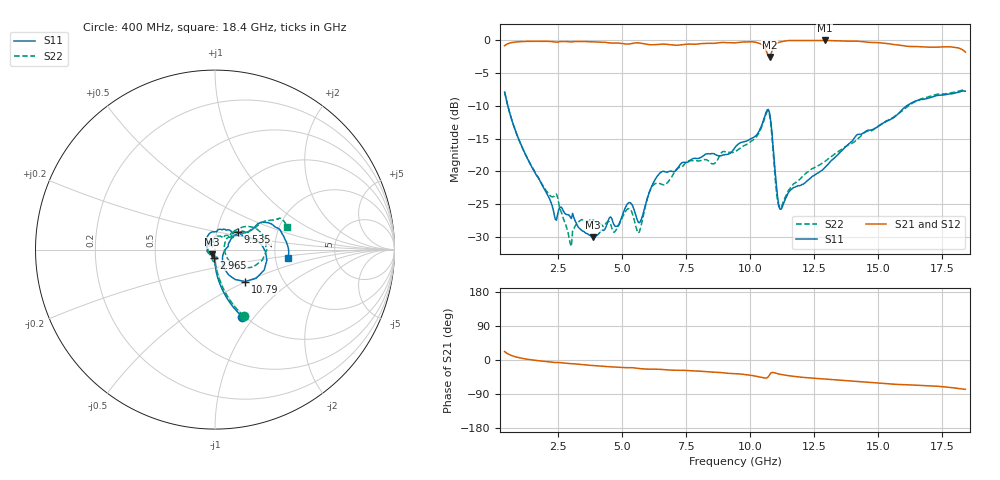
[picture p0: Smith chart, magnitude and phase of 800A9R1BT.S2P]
!  American Technical Ceramics  Date:  12/17/08
!  One Norden Lane
!  Huntington Station,  NY.  11746-2102
!  Tel:  (631) 622-4700  Fax:  (631) 622-4748
!  Part Number  800A9R1BT
!  Description: Broardband capacitor  Mounting Orientation: Vertical
!  Application:
# GHZ S DB R 50
! Freq  |S11|  S11 Ph  |S21|  S21 Ph  |S12|  S12 Ph  |S22|  S22 Ph
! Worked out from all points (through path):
!   401 points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, 400 MHz to 18.4 GHz, reference 50 ohm
!   highest |S21| = 0.00 dB at 12.91 GHz (marker M1); lowest = -2.5 dB at 10.75 GHz (marker M2)
!   group delay of S21, straight-line fit = 12.2 ps
!   lowest |S11| = -30.1 dB at 3.865 GHz (marker M3), VSWR 1.06, Z = 48.2 - j2.5 ohm
!   |S11| at or under -10 dB: 525.5 MHz to 16.1 GHz (15.58 GHz wide, 187 % of centre)
!   |S22| runs from -31.5 to -7.5 dB; largest |S21 - S12| = 0.0018
!   S11 on the Smith chart (normalised r, x): 400 MHz: 0.97, -0.87; 2.965 GHz: 0.99, -0.09; 9.535 GHz: 1.27, +0.25; 10.79 GHz: 1.30, -0.49; 18.4 GHz: 2.35, -0.26
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0.4  -7.89 -67.9  -0.81 22.1  -0.81 22.1  -7.88 -66.7
1.255  -17.76 -86.4  -0.14 2.3  -0.14 2.3  -17.76 -84.3
2.335  -26.52 -91.3  -0.22 -6.5  -0.21 -6.5  -23.83 -89.2
2.965  -26.99 -96.8  -0.22 -9.6  -0.21 -9.6  -31.06 -105.2
3.415  -29.06 -110.2  -0.16 -12.2  -0.15 -12.2  -27.39 -105.3
3.865  -30.10 -124.2  -0.21 -14.7  -0.21 -14.7  -27.50 -126.1
4.72  -28.43 175.4  -0.39 -18.6  -0.38 -18.6  -29.18 -169.3
5.26  -24.80 142.8  -0.54 -20.1  -0.54 -20.2  -25.71 130.2
5.62  -27.78 124.0  -0.37 -22.2  -0.37 -22.2  -29.46 100.3
6.07  -23.05 130.4  -0.65 -24.1  -0.64 -24.1  -23.02 87.6
6.43  -20.44 108.7  -0.60 -24.5  -0.60 -24.5  -21.85 59.6
9.4  -16.38 40.3  -0.37 -36.1  -0.37 -36.2  -16.99 42.6
9.535  -15.83 36.5  -0.32 -36.6  -0.32 -36.6  -16.68 43.9
10.435  -13.05 15.4  -0.61 -45.7  -0.61 -45.7  -13.29 36.5
10.75  -11.09 -35.0  -2.53 -39.0  -2.52 -39.0  -11.38 -12.7
10.795  -12.25 -46.9  -2.19 -34.9  -2.19 -34.9  -12.63 -24.6
11.02  -22.27 -57.0  -0.48 -35.3  -0.48 -35.4  -23.21 -27.9
11.155  -25.81 -26.8  -0.24 -37.7  -0.24 -37.7  -25.59 4.2
12.415  -20.80 27.5  -0.01 -47.8  -0.01 -47.8  -19.60 41.1
12.91  -19.44 33.8  0.00 -50.5  -0.01 -50.5  -18.52 38.2
15.43  -12.15 28.8  -0.52 -63.2  -0.51 -63.2  -12.07 28.1
18.4  -7.76 -6.3  -1.78 -77.3  -1.78 -77.3  -7.54 17.3
